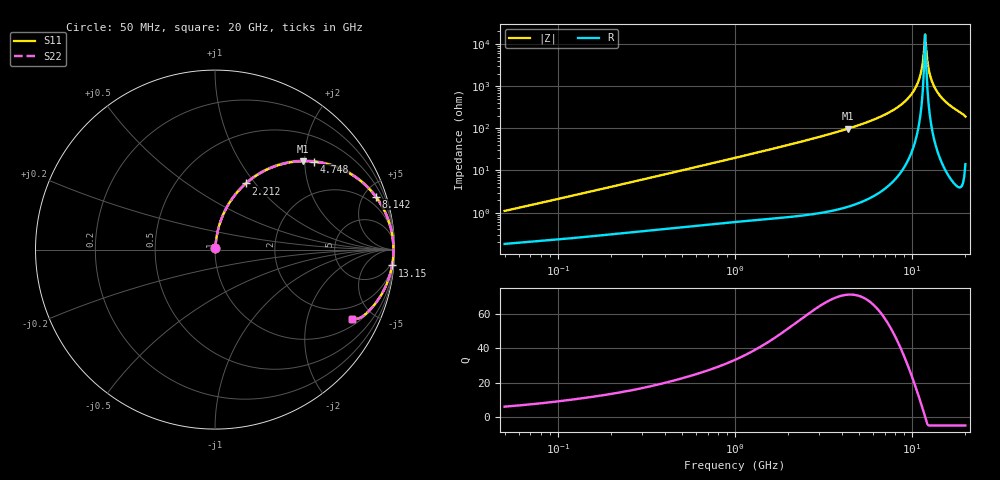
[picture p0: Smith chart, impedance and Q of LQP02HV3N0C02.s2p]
!Murata Part Number: LQP02HV3N0C02
!These Parameters are Measured in Series Mode Connection
!  o--[Z]--o
!Port1  Port2
!  o-------o
!Freq. Start=50[MHz] Stop=20[GHz], 401[Steps]
# Hz S RI R 50
!Freq.(Hz) S11(Real) S11(Imag) S21(Real) S21(Imag) S12(Real) S12(Imag) S22(Real) S22(Imag)
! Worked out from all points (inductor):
!   401 points, 50 MHz to 20 GHz, reference 50 ohm
!   read as one part in series: L = 3.4 nH near 51.52 MHz
!   highest Q = 71.4 at 4.34 GHz (marker M1), where L = 3.59 nH
!   self-resonance near 11.84 GHz
!   S11 on the Smith chart (normalised r, x): 50 MHz: 1.00, +0.02; 2.212 GHz: 1.02, +0.90; 4.748 GHz: 1.03, +2.21; 8.142 GHz: 1.13, +6.02; 13.15 GHz: 2, -22; 20 GHz: 1.28, -3.78
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5e7  0.00192 0.0108  0.9981 -0.0108  0.9981 -0.0108  0.00192 0.0108
1.364002e8  0.00339 0.0281  0.9966 -0.0281  0.9966 -0.0281  0.00339 0.0281
3.721004e8  0.00943 0.0739  0.9906 -0.0739  0.9906 -0.0739  0.00943 0.0739
1e9  0.0434 0.1892  0.9566 -0.1892  0.9566 -0.1892  0.0434 0.1892
2.211938e9  0.1724 0.3688  0.8276 -0.3688  0.8276 -0.3688  0.1724 0.3688
2.728004e9  0.245 0.4221  0.755 -0.4221  0.755 -0.4221  0.245 0.4221
4.34015e9  0.4902 0.4929  0.5098 -0.4929  0.5098 -0.4929  0.4902 0.4929
4.748272e9  0.5495 0.4906  0.4505 -0.4906  0.4505 -0.4906  0.5495 0.4906
7.442007e9  0.8473 0.3504  0.1527 -0.3504  0.1527 -0.3504  0.8473 0.3504
8.141811e9  0.8954 0.2953  0.1046 -0.2953  0.1046 -0.2953  0.8954 0.2953
9.457416e9  0.9568 0.1872  0.0432 -0.1872  0.0432 -0.1872  0.9568 0.1872
1.050288e10  0.9832 0.1026  0.0168 -0.1026  0.0168 -0.1026  0.9832 0.1026
1.098561e10  0.9898 0.0649  0.0102 -0.0649  0.0102 -0.0649  0.9898 0.0649
1.131968e10  0.9925 0.0395  0.00747 -0.0395  0.00747 -0.0395  0.9925 0.0395
1.149051e10  0.9934 0.0267  0.00658 -0.0267  0.00658 -0.0267  0.9934 0.0267
1.183995e10  0.9942 0.00111  0.00579 -0.00111  0.00579 -0.00111  0.9942 0.00111
1.220001e10  0.9937 -0.0245  0.00632 0.0245  0.00632 0.0245  0.9937 -0.0245
1.257102e10  0.9918 -0.0501  0.00818 0.0501  0.00818 0.0501  0.9918 -0.0501
1.314879e10  0.9866 -0.0882  0.0134 0.0882  0.0134 0.0882  0.9866 -0.0882
1.396067e10  0.975 -0.1381  0.025 0.1381  0.025 0.1381  0.975 -0.1381
1.527346e10  0.9481 -0.2099  0.0519 0.2099  0.0519 0.2099  0.9481 -0.2099
2e10  0.766 -0.3876  0.234 0.3876  0.234 0.3876  0.766 -0.3876
